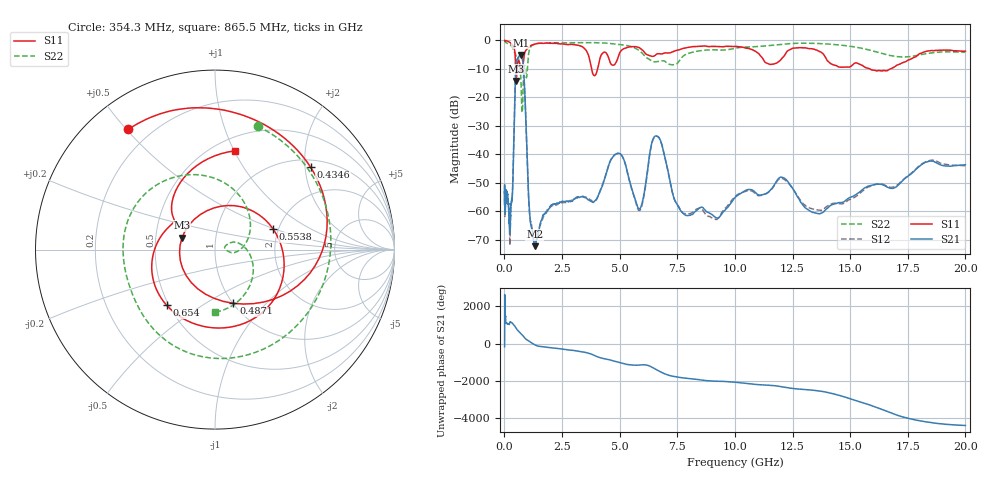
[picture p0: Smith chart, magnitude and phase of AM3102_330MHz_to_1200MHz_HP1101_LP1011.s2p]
! Date/Time: Tue, Sep 11, 2018 5:22 PM
! Network Analyzer: Agilent Technologies E8362B Rev: A.07.50.63
! Sweep from 0.010 to 20.000 GHz, 1601 Points, Sweep Type: LOG
! Power Supply: 4.949 V, 0.001 A
# Hz S DB R 50
!freq MagS11 AngS11 MagS21 AngS21 MagS12 AngS12 MagS22 AngS22
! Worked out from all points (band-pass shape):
!   1601 points, 10 MHz to 20 GHz, reference 50 ohm
!   highest |S21| = -5.10 dB at 712.4 MHz (marker M1); lowest = -72.2 dB at 1.321 GHz (marker M2)
!   |S21| within 3 dB of the highest: 512.6 MHz to 809.7 MHz (297.1 MHz wide, 44.9 % of centre)
!   lowest |S11| = -14.2 dB at 513.3 MHz (marker M3), VSWR 1.49, Z = 34.2 + j4.79 ohm
!   |S11| at or under -10 dB: 710.3 MHz to 789.6 MHz (79.31 MHz wide, 10.6 % of centre); 3.787 GHz to 4.043 GHz (256.6 MHz wide, 6.56 % of centre); 15.86 GHz to 16.75 GHz (890.1 MHz wide, 5.46 % of centre)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
!   |S22| runs from -25.2 to -0.2 dB; largest |S21 - S12| = 0.0092
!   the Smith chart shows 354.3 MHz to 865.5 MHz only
!   S11 on the Smith chart (normalised r, x): 354.3 MHz: 0.12, +0.51; 434.6 MHz: 1.18, +2.14; 487.1 MHz: 1.01, -0.67; 553.8 MHz: 1.87, +0.49; 654 MHz: 0.49, -0.36; 865.5 MHz: 0.63, +1.01
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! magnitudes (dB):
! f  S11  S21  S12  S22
! 10 MHz  0.0  -53.8  -50.3  -0.2
! 35.55 MHz  -0.1  -59.7  -58.3  -0.5
! 126.4 MHz  -0.2  -53.6  -53.8  -1.0
! 240 MHz  -0.7  -66.3  -71.3  -1.4
! 354.3 MHz  -1.7  -53.0  -52.7  -2.8
! 434.6 MHz  -3.1  -26.0  -26.0  -4.1
! 447.2 MHz  -3.6  -22.0  -22.1  -4.2
! 487.1 MHz  -10.0  -11.6  -11.6  -5.0
! 513.3 MHz  -14.2  -8.0  -8.2  -5.6
! 553.8 MHz  -9.3  -6.6  -6.6  -5.8
! 654 MHz  -7.7  -5.4  -5.5  -8.1
! 712.4 MHz  -10.1  -5.1  -5.1  -13.2
! 772.3 MHz  -10.8  -6.0  -6.0  -25.2
! 865.5 MHz  -5.0  -14.8  -15.0  -9.1
! 1.082 GHz  -2.2  -59.1  -59.7  -3.5
! 1.321 GHz  -1.3  -72.2  -70.8  -1.3
! 1.59 GHz  -1.0  -63.3  -64.0  -1.0
! 4.902 GHz  -6.7  -39.6  -39.7  -1.4
! 5.652 GHz  -2.2  -55.2  -55.4  -2.6
! 6.612 GHz  -4.8  -33.6  -33.6  -7.5
! 7.958 GHz  -2.5  -61.5  -60.9  -4.6
! 20 GHz  -3.8  -43.6  -44.0  -4.1
